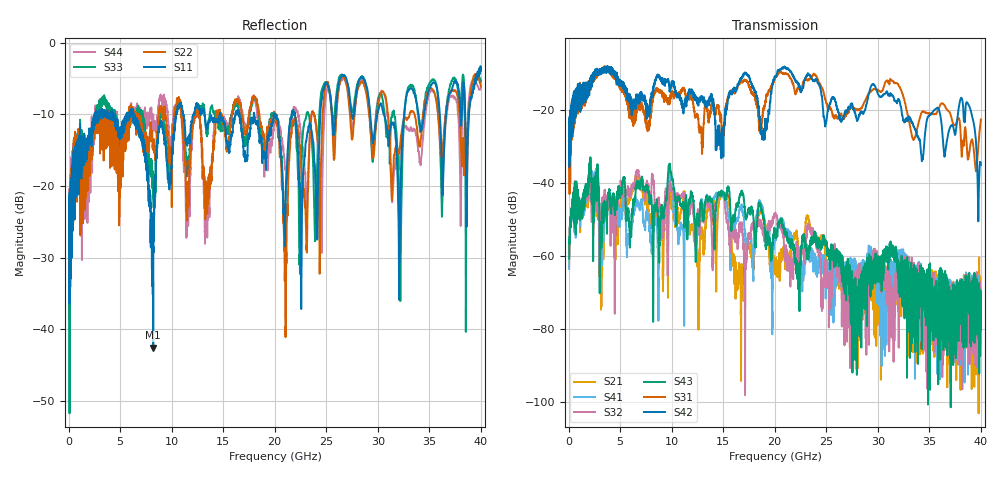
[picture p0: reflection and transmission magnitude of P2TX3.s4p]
!Agilent Technologies,N5245A,MY49151084,A.09.20.08
!Agilent N5245A: A.09.20.08
!Date: Thursday, March 01, 2012 14:26:11
!Correction: S11(Full 4 Port(1,2,3,4))
!S12(Full 4 Port(1,2,3,4))
!S13(Full 4 Port(1,2,3,4))
!S14(Full 4 Port(1,2,3,4))
!S21(Full 4 Port(1,2,3,4))
!S22(Full 4 Port(1,2,3,4))
!S23(Full 4 Port(1,2,3,4))
!S24(Full 4 Port(1,2,3,4))
!S31(Full 4 Port(1,2,3,4))
!S32(Full 4 Port(1,2,3,4))
!S33(Full 4 Port(1,2,3,4))
!S34(Full 4 Port(1,2,3,4))
!S41(Full 4 Port(1,2,3,4))
!S42(Full 4 Port(1,2,3,4))
!S43(Full 4 Port(1,2,3,4))
!S44(Full 4 Port(1,2,3,4))
!S4P File: Measurements: <S11,S12,S13,S14>,
!<S21,S22,S23,S24>,
!<S31,S32,S33,S34>,
!<S41,S42,S43,S44>:
# Hz S  dB  R 50
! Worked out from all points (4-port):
!   3996 points, 50 MHz to 40 GHz, reference 50 ohm
!   strongest paths, dB at 50 MHz, 10.04 GHz, 20.03 GHz, 30.02 GHz, 40 GHz:
!     S42: -24.6, -12.8, -10.9, -15.6, -35.0
!     S31: -25.5, -15.5, -11.2, -14.4, -22.6
!     S43: -60.7, -38.6, -52.8, -64.0, -72.3
!     S32: -57.0, -41.4, -48.4, -64.0, -70.5
!     S41: -63.5, -42.8, -54.8, -69.2, -74.7
!     S21: -63.0, -45.4, -64.9, -64.9, -73.4
!   lowest |S11| = -42.6 dB at 8.21 GHz (marker M1), VSWR 1.02, Z = 49.9 - j0.737 ohm
!   |S11| at or under -10 dB: start of sweep to 2.53 GHz; 6.361 GHz to 10.45 GHz (4.085 GHz wide, 48.6 % of centre); 21.97 GHz to 24.42 GHz (2.454 GHz wide, 10.6 % of centre)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
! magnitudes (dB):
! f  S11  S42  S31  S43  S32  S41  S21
! 50 MHz  -23.3  -24.6  -25.5  -60.7  -57.0  -63.5  -63.0
! 2.03 GHz  -12.2  -12.9  -12.0  -36.4  -37.7  -36.5  -37.7
! 8.21 GHz  -42.6  -14.1  -16.6  -69.6  -39.1  -53.3  -48.4
! 21.03 GHz  -22.7  -8.3  -9.9  -53.1  -59.6  -54.0  -63.5
! 25.07 GHz  -5.6  -21.5  -18.3  -58.4  -66.0  -63.0  -64.5
! 32.07 GHz  -35.9  -17.4  -13.5  -65.5  -73.4  -63.6  -67.0
! 40 GHz  -3.9  -35.0  -22.6  -72.3  -70.5  -74.7  -73.4
